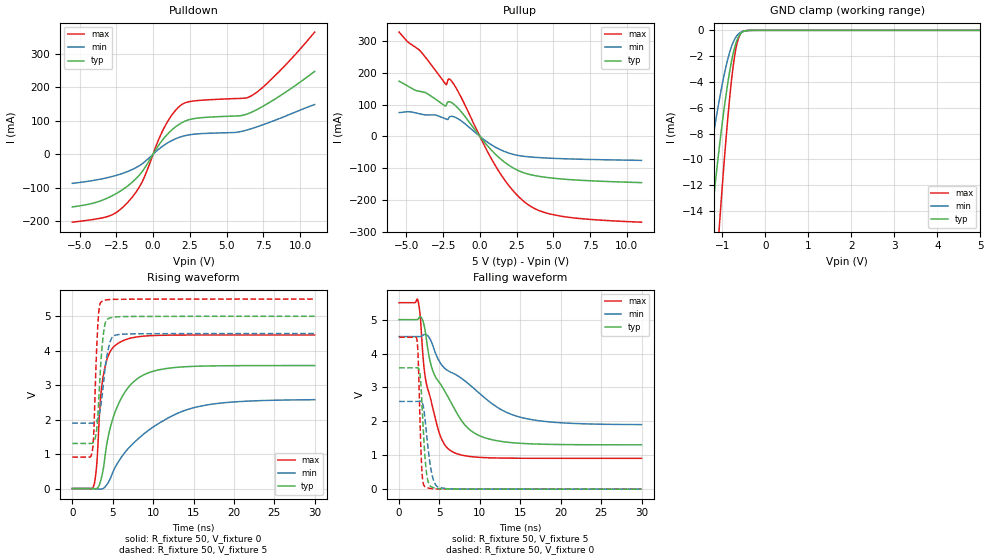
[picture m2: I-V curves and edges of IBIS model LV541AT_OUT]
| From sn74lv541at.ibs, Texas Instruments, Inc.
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[Model]   LV541AT_OUT
Model_type  3-state
Enable   Active-Low
Vref =   0
Rref =   1000
Cref =   50p
Vmeas =   1.5
| variable   typ   min   max
C_comp   4.12pF   3.11pF   4.82pF
| C_pullup   6.84pF   3.28pF   11.40pF
| C_pulldown   6.78pF   3.86pF   11.60pF
| C_tri-state   4.12pF   3.11pF   4.82pF
[Temperature Range]   40   100   -40
| Ambient temperature   25   85   -40
[Voltage range]   5   4.5   5.5
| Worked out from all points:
|   slope of the pulldown table from 0 to 0.75 V, typ, clamps not added: 15.5 ohm
|   slope of the pullup table from 0 to 0.75 V, typ, clamps not added: 18 ohm
|   GND clamp passes 1 mA (typ) near -0.69 V on its own axis
|   rising waveform, R_fixture 50, V_fixture 0: 20-80 % time 2.75ns typ, 6.89ns min, 1ns max; typ from 0 V to 3.57 V
|   falling waveform, R_fixture 50, V_fixture 5: 20-80 % time 4.18ns typ, 7.54ns min, 1.99ns max; typ from 5 V to 1.31 V
|   rising waveform, R_fixture 50, V_fixture 5: 20-80 % time 606ps typ, 848ps min, 428ps max; typ from 1.31 V to 5 V
|   falling waveform, R_fixture 50, V_fixture 0: 20-80 % time 533ps typ, 786ps min, 343ps max; typ from 3.58 V to 0 V
[GND Clamp]
| LV541AT_OUT
|   Voltage   I(typ)   I(min)   I(max)
-5.5V     -228mA     -149.7mA   -287mA
-1.54V    -24.85mA   -15.68mA   -39.41mA
-1.485V   -22.78mA   -14.34mA   -36.39mA
-1.26V    -14.88mA   -9.182mA   -24.47mA
-1.08V    -9.319mA   -5.552mA   -15.62mA
-1.055V   -8.61mA    -5.091mA   -14.46mA
-910mV    -4.881mA   -2.716mA   -8.194mA
-840mV    -3.372mA   -1.805mA   -5.572mA
-765mV    -2.035mA   -1.051mA   -3.212mA
-655mV    -716.1uA   -380.9uA   -950.6uA
-545mV    -149.8uA   -102.8uA   -148.9uA
5V        66.21nA    4.462nA    635.2nA
[Pulldown]
| LV541AT_OUT
|   Voltage   I(typ)   I(min)   I(max)
-5.5V     -157.8mA   -87.14mA   -203.3mA
-2.975V   -128.4mA   -68.75mA   -184.5mA
-1.725V   -94.85mA   -51.6mA    -144mA
-725mV    -50.87mA   -28.07mA   -81.03mA
335mV     23.73mA    13.24mA    39.13mA
835mV     52.74mA    29.57mA    85.85mA
1.865V    91.83mA    51.57mA    145.6mA
2.82V     106.7mA    60.04mA    159.5mA
5.62V     114.3mA    65.19mA    166.4mA
6.675V    125mA      76.05mA    174.2mA
8.565V    172.3mA    106.1mA    246.3mA
11V       247.6mA    148.4mA    365.1mA
[Pullup]
| LV541AT_OUT
|   Voltage   I(typ)   I(min)   I(max)
-5.5V     173.7mA    74.89mA    328.5mA
-4.9V     158.2mA    77.67mA    297.3mA
-4.045V   141.3mA    70.44mA    268.3mA
-2.31V    95.97mA    54.84mA    163.4mA
-2.115V   109.2mA    58.62mA    180.8mA
-1.885V   105.1mA    63.04mA    171.6mA
1.105V    -58.37mA   -35.22mA   -96.24mA
2.105V    -94.93mA   -54.59mA   -162.7mA
3.09V     -116.2mA   -63.24mA   -208.5mA
4.085V    -126.3mA   -66.98mA   -234.7mA
5.505V    -134mA     -70.14mA   -251.2mA
11V       -145.6mA   -75.58mA   -270.3mA
[Ramp]
| LV541AT_OUT
| variable   typ   min   max
dV/dt_r   2.15/2.75E-09   1.56/6.88E-09   2.68/1.01E-09
dV/dt_f   2.27/4.18E-09   1.60/7.54E-09   2.82/1.99E-09
R_load = 50
[Rising Waveform]
| LV541AT_OUT
R_fixture =   50
C_fixture =   0
L_fixture =   0
V_fixture =   0
V_fixture_min = 0
V_fixture_max = 0
|   Time   V(typ)   V(min)   V(max)
0s        1.266nV    819pV      2.497nV
2.69ns    -13.36mV   -900.6uV   103.5mV
3.03ns    1.994mV    -8.544mV   704.7mV
3.46ns    183.7mV    -18.7mV    2.504V
3.85ns    588mV      6.12mV     3.294V
4.61ns    1.678V     242.3mV    3.941V
5.725ns   2.458V     782.1mV    4.222V
8.67ns    3.279V     1.549V     4.42V
14.32ns   3.54V      2.298V     4.456V
29.99ns   3.569V     2.579V     4.457V
[Falling Waveform]
| LV541AT_OUT
R_fixture =   50
C_fixture =   0
L_fixture =   0
V_fixture =   5
V_fixture_min = 4.5
V_fixture_max = 5.5
|   Time   V(typ)   V(min)   V(max)
0s        5V         4.5V       5.5V
2.31ns    5.012V     4.499V     5.586V
2.875ns   5.007V     4.527V     4.19V
3.395ns   4.401V     4.553V     3.097V
4.25ns    3.442V     4.186V     2.312V
6.41ns    2.564V     3.449V     1.13V
8.59ns    1.785V     3.107V     969.4mV
11.53ns   1.457V     2.516V     922.4mV
17.12ns   1.33V      2.024V     910.9mV
29.99ns   1.308V     1.903V     910.3mV
[Rising Waveform]
| LV541AT_OUT
R_fixture =   50
C_fixture =   0
L_fixture =   0
V_fixture =   5
V_fixture_min = 4.5
V_fixture_max = 5.5
|   Time   V(typ)   V(min)   V(max)
0s        1.308V     1.898V     910.3mV
2.445ns   1.314V     1.896V     1.043V
2.655ns   1.358V     1.898V     1.6V
2.975ns   1.632V     1.945V     3.807V
3.19ns    2.213V     2.038V     4.853V
3.675ns   4.074V     2.655V     5.435V
4.025ns   4.745V     3.419V     5.467V
4.42ns    4.927V     4.01V      5.482V
5.305ns   4.98V      4.45V      5.492V
29.99ns   5V         4.5V       5.5V
[Falling Waveform]
| LV541AT_OUT
R_fixture =   50
C_fixture =   0
L_fixture =   0
V_fixture =   0
V_fixture_min = 0
V_fixture_max = 0
|   Time   V(typ)   V(min)   V(max)
0s        3.579V     2.588V     4.481V
2.205ns   3.582V     2.588V     4.415V
2.37ns    3.572V     2.59V      3.825V
2.6ns     3.358V     2.595V     1.938V
2.795ns   2.686V     2.577V     658.6mV
3.205ns   951.2mV    2.078V     73.38mV
3.545ns   266.8mV    1.296V     38.76mV
4.03ns    64.25mV    474.1mV    14.83mV
4.955ns   14.69mV    54.81mV    3.864mV
29.99ns   1.44uV     13.15uV    7.112nV
